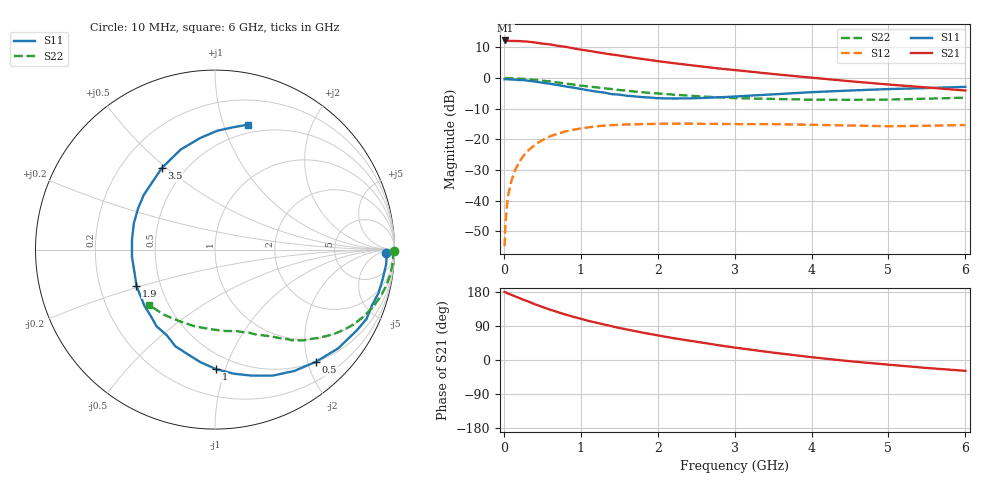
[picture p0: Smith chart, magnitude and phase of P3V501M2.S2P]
! SIEMENS Small Signal Semiconductors
! BFP181
! Si NPN RF Bipolar Junction Transistor in SOT143
! VCE = 0.5 V  IC = 1.2 mA
! Common Emitter S-Parameters:  March  1996
# GHz  S  MA  R  50
!  f  S11  S21  S12  S22
! GHz  MAG  ANG  MAG  ANG  MAG  ANG  MAG  ANG
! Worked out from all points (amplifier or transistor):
!   36 points, 10 MHz to 6 GHz, reference 50 ohm
!   highest |S21| = 12.3 dB at 20 MHz (marker M1)
!   |S21| within 3 dB of that: start of sweep to 997.9 MHz
!   unconditionally stable (mu >= 1): 2.508 GHz to end of sweep
!   at 250 MHz: K = 0.11, MSG = 18.8 dB, |S12| = -25.6 dB
!   at 1.4 GHz: K = 0.60, MSG = 11.5 dB, |S12| = -15.4 dB
!   at 6 GHz: K = 1.48, MAG = 1.6 dB, |S12| = -15.3 dB
!   S11 on the Smith chart (normalised r, x): 10 MHz: 38, -15; 500 MHz: 0.50, -2.15; 1 GHz: 0.39, -0.93; 1.9 GHz: 0.36, -0.19; 3.5 GHz: 0.37, +0.48; 6 GHz: 0.42, +1.21
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0.01  0.9553 -1.0  4.081 179.5  0.0018 93.2  0.9968 -0.4
0.02  0.9571 -2.1  4.118 178.9  0.0041 88.6  0.9903 -1.0
0.05  0.9573 -4.8  4.081 175.9  0.0113 88.3  0.9931 -2.6
0.1  0.9488 -9.9  4.039 171.9  0.0215 84.0  0.9919 -5.1
0.15  0.9428 -14.8  4.036 167.6  0.0321 79.7  0.986 -7.8
0.3  0.9101 -29.5  3.954 155.8  0.0629 70.8  0.9616 -15.1
0.4  0.8797 -38.7  3.821 147.5  0.0809 64.9  0.9372 -19.9
0.5  0.841 -48.0  3.656 139.9  0.097 58.9  0.9078 -24.2
0.6  0.8075 -56.9  3.548 133.0  0.112 53.7  0.8799 -28.1
0.8  0.7317 -73.7  3.247 120.0  0.1344 44.4  0.8174 -34.8
1  0.6653 -89.6  2.912 108.8  0.1504 36.5  0.7556 -40.7
1.1  0.6328 -97.3  2.798 103.2  0.1572 33.0  0.7286 -43.1
1.3  0.5817 -112.4  2.54 93.8  0.1671 26.6  0.684 -47.6
1.5  0.537 -127.4  2.337 84.6  0.1722 21.6  0.6392 -51.2
1.9  0.4813 -155.4  1.974 68.7  0.178 13.3  0.5721 -57.7
2.2  0.4644 -175.1  1.758 57.8  0.1803 8.8  0.5382 -62.2
2.8  0.4863 151.8  1.433 38.7  0.1787 1.6  0.4861 -71.2
3.5  0.5423 123.2  1.166 19.5  0.1771 -3.9  0.4566 -83.2
4  0.5891 109.0  1.016 7.4  0.1727 -7.1  0.4437 -93.8
4.5  0.6268 97.7  0.888 -3.3  0.1682 -9.5  0.4421 -105.3
5.5  0.688 81.8  0.703 -21.1  0.1665 -9.2  0.4613 -128.2
6  0.7195 75.3  0.627 -28.6  0.1713 -9.3  0.479 -139.7
